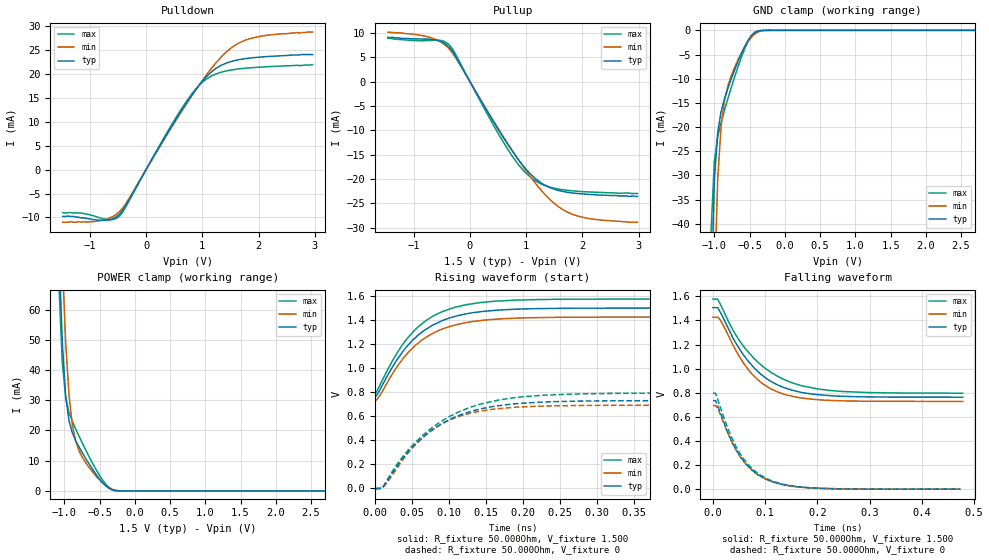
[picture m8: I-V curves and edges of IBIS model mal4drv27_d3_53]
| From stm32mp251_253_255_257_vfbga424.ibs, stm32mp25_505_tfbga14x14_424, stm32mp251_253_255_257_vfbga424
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[Model] mal4drv27_d3_53
Model_type   I/O
Polarity   Non-Inverting
Enable   Active-High
C_comp   1.653pF   1.649pF   1.658pF
C_comp_pullup   821.240fF   815.174fF   828.427fF
C_comp_pulldown 737.945fF   733.914fF   744.436fF
Vinh = 885.000mV
Vinl = 615.000mV
Vmeas = 750.000mV
Vref = 750.000mV
Rref = 50Ohms
Cref = 0pF
[Model Spec]
Vinh   885.000mV   848.000mV   923.000mV
Vinl   615.000mV   578.000mV   653.000mV
Vmeas   750.000mV   713.000mV   788.000mV
Vref   750.000mV   713.000mV   788.000mV
D_overshoot_ampl_h 0.4 NA   NA
D_overshoot_ampl_l 0.4 NA   NA
D_overshoot_area_l 100.000m NA   NA
D_overshoot_area_h 100.000m NA   NA
[Receiver Thresholds]
Vth = 750.000mV
Vth_min = 713.000mV
Vth_max = 788.000mV
Vinh_ac = 135.000mV
Vinh_dc = 100.000mV
Vinl_ac = -135.000mV
Vinl_dc = -100.000mV
Tslew_ac = 5.000ns
Threshold_sensitivity = 0.5
Reference_supply Pullup_ref
[Temperature Range]   25.000   125.000   -40.000
[Voltage Range]   1.500V   1.425V   1.575V
[GND Clamp Reference]   0.00V   0.00V   0.00V
[C Comp Corner]
| variable   typ   min   max
C_comp 1.658pF   1.653pF   1.649pF
C_comp_pullup 821.240fF   828.427fF   815.174fF
C_comp_pulldown 733.914fF   744.436fF   737.945fF
[Pulldown Reference]   0.00V   0.00V   0.00V
[POWER Clamp Reference]   1.500V   1.425V   1.575V
[Pullup Reference]   1.500V   1.425V   1.575V
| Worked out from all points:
|   slope of the pulldown table from 0 to 0.225 V, typ, clamps not added: 49.2 ohm
|   slope of the pullup table from 0 to 0.225 V, typ, clamps not added: 50.1 ohm
|   GND clamp passes 1 mA (typ) near -0.47 V on its own axis
|   POWER clamp passes 1 mA (typ) near -0.37 V on its own axis
|   rising waveform, R_fixture 50.000Ohm, V_fixture 1.500: 20-80 % time 62.1ps typ, 61.5ps min, 60.8ps max; typ from 0.758 V to 1.5 V
|   rising waveform, R_fixture 50.000Ohm, V_fixture 0: 20-80 % time 79.4ps typ, 69.2ps min, 87.3ps max; typ from -0.001 V to 0.729 V
|   falling waveform, R_fixture 50.000Ohm, V_fixture 1.500: 20-80 % time 78ps typ, 69.6ps min, 90.8ps max; typ from 1.51 V to 0.763 V
|   falling waveform, R_fixture 50.000Ohm, V_fixture 0: 20-80 % time 60.1ps typ, 59.7ps min, 60.6ps max; typ from 0.734 V to 0 V
[GND Clamp]
-1.48V    -1.356A    -1.372A    -1.368A
-1.05V    -57.52mA   -98.82mA   -41.99mA
-1.002V   -31.12mA   -53.93mA   -27.05mA
-954.6mV  -21.13mA   -30.8mA    -21.99mA
-906.8mV  -16.83mA   -19.93mA   -19.06mA
-859.1mV  -14.2mA    -14.62mA   -16.56mA
-763.6mV  -10.09mA   -9.457mA   -11.91mA
-668.2mV  -6.482mA   -6.16mA    -7.611mA
-525mV    -2.097mA   -2.366mA   -2.333mA
-429.5mV  -449.8uA   -771.1uA   -394uA
-238.6mV  -1.709uA   -14.74uA   -370nA
2.959V    53.06nA    707.1nA    76.78nA
[Power Clamp]
-1.459V   570.2mA    591.8mA    567.2mA
-1.077V   80.71mA    114.2mA    68.27mA
-1.03V    49.21mA    76.71mA    42.66mA
-981.8mV  31.4mA     49.26mA    30.9mA
-934.1mV  23.16mA    31.72mA    25.95mA
-886.4mV  19.16mA    21.79mA    22.98mA
-838.6mV  16.6mA     16.39mA    20.46mA
-743.2mV  12.52mA    11.03mA    15.74mA
-647.7mV  8.857mA    7.696mA    11.27mA
-361.4mV  773.2uA    986uA      1.034mA
-218.2mV  12.39uA    63.5uA     9.952uA
2.98V     -55.08nA   -1.144uA   -55.82nA
[Pulldown]
-1.48V    -9.8mA     -11mA      -9mA
-1.145V   -10.1mA    -11mA      -9.1mA
-763.6mV  -10.62mA   -10.57mA   -10.3mA
-477.3mV  -9.369mA   -8.839mA   -9.77mA
-334.1mV  -6.932mA   -6.645mA   -7.244mA
286.4mV   5.801mA    5.64mA     6.028mA
715.9mV   13.92mA    13.73mA    14.26mA
954.6mV   17.84mA    17.9mA     17.78mA
1.241V    21.18mA    22.35mA    20.02mA
1.527V    22.7mA     25.62mA    20.89mA
1.814V    23.31mA    27.31mA    21.28mA
2.959V    24.1mA     28.8mA     22mA
[Pullup]
-1.459V   9.1mA      10.2mA     8.957mA
-743.2mV  8.75mA     9.21mA     8.469mA
-504.6mV  8.206mA    8.05mA     8.456mA
-361.4mV  6.985mA    6.638mA    7.493mA
-265.9mV  5.396mA    5.158mA    5.869mA
640.9mV   -12.35mA   -12.15mA   -13.34mA
927.3mV   -17.03mA   -17.16mA   -17.97mA
1.166V    -19.95mA   -20.92mA   -20.4mA
1.5V      -22.11mA   -25.05mA   -21.91mA
1.834V    -22.91mA   -27.32mA   -22.46mA
2.264V    -23.29mA   -28.38mA   -22.75mA
2.98V     -23.6mA    -28.9mA    -23mA
[Ramp]
R_load=50.000Ohm
dV/dt_r   439.920mV/71.500ps  416.488mV/66.000ps  471.270mV/75.500ps
dV/dt_f   439.920mV/70.000ps  416.488mV/65.500ps  471.270mV/77.000ps
[Rising waveform]
R_fixture=50.000Ohm
V_fixture=1.500
V_fixture_min=1.425
V_fixture_max=1.575
0s        758.2mV    727.6mV    787.4mV
6ps       817.1mV    770.5mV    856.6mV
29ps      1.067V     1.008V     1.122V
49ps      1.223V     1.159V     1.289V
60ps      1.286V     1.219V     1.355V
75ps      1.349V     1.28V      1.422V
108ps     1.431V     1.359V     1.507V
145ps     1.472V     1.398V     1.548V
196ps     1.492V     1.417V     1.567V
469ps     1.5V       1.425V     1.575V
[Rising waveform]
R_fixture=50.000Ohm
V_fixture=0
0s        -1.396mV   -1.68mV    -8.148mV
10ps      6.235mV    3.998mV    9.439mV
41ps      275.5mV    268mV      292.4mV
58ps      387.1mV    387.3mV    405.1mV
76ps      480.1mV    481.9mV    500.2mV
103ps     579mV      574.3mV    605.7mV
141ps     658.6mV    640.6mV    698.3mV
184ps     700.1mV    671.6mV    750.9mV
241ps     720.3mV    685.7mV    778.6mV
478ps     729.2mV    691mV      791.8mV
[Falling waveform]
R_fixture=50.000Ohm
V_fixture=1.500
V_fixture_min=1.425
V_fixture_max=1.575
0s        1.506V     1.426V     1.577V
9ps       1.506V     1.426V     1.577V
13ps      1.478V     1.409V     1.545V
43ps      1.218V     1.158V     1.285V
74ps      1.029V     959.3mV    1.106V
101ps     922.4mV    857.5mV    999.7mV
131ps     850.6mV    795mV      919.6mV
170ps     802.1mV    756mV      857.8mV
244ps     771.2mV    733.2mV    811.2mV
478ps     763mV      727.9mV    796.2mV
[Falling waveform]
R_fixture=50.000Ohm
V_fixture=0
0s        734.5mV    693.1mV    796.1mV
5ps       734.5mV    693.1mV    796.1mV
8ps       705.6mV    679.5mV    761.3mV
32ps      434.5mV    430.8mV    468.2mV
55ps      254.8mV    252.3mV    275.3mV
82ps      133.3mV    132mV      144.7mV
113ps     63.2mV     62.27mV    68.25mV
154ps     23.57mV    22.92mV    25.18mV
200ps     7.572mV    7.405mV    7.987mV
474ps     5.908uV    14.4uV     8.796uV
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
